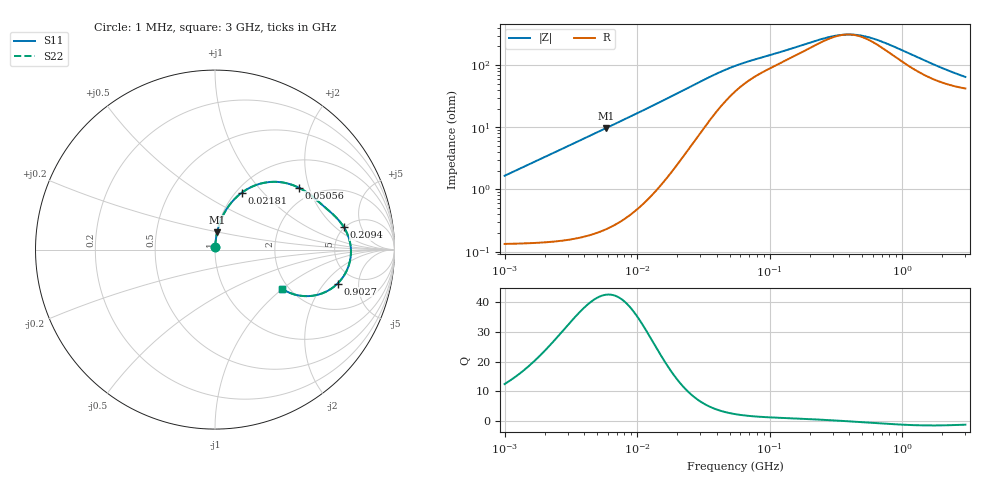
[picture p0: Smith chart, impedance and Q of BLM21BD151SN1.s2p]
! BLM21BD151SN1
# Hz S RI R 50
!Freq.(Hz) S11(Real) S11(Imag) S21(Real) S21(Imag) S12(Real) S12(Imag) S22(Real) S22(Imag)
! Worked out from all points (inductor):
!   401 points, 1 MHz to 3 GHz, reference 50 ohm
!   read as one part in series: L = 263 nH near 1.041 MHz
!   highest Q = 42.5 at 5.821 MHz (marker M1), where L = 265 nH
!   self-resonance near 385.4 MHz
!   S11 on the Smith chart (normalised r, x): 1 MHz: 1.00, +0.03; 21.81 MHz: 1.06, +0.77; 50.56 MHz: 1.64, +1.71; 209.4 MHz: 4.95, +2.62; 902.7 MHz: 3.65, -2.77; 3 GHz: 1.84, -0.98
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1000000  0.0016 0.0165  0.9984 -0.0165  0.9984 -0.0165  0.0016 0.0165
3823119  0.00568 0.0629  0.9943 -0.0629  0.9943 -0.0629  0.00568 0.0629
5820586  0.0115 0.0955  0.9885 -0.0955  0.9885 -0.0955  0.0115 0.0955
9410094  0.0283 0.1528  0.9717 -0.1528  0.9717 -0.1528  0.0283 0.1528
1.461624e7  0.0676 0.2305  0.9324 -0.2305  0.9324 -0.2305  0.0676 0.2305
2.181181e7  0.1484 0.3164  0.8516 -0.3164  0.8516 -0.3164  0.1484 0.3164
2.773354e7  0.2281 0.3596  0.7719 -0.3596  0.7719 -0.3596  0.2281 0.3596
3.387922e7  0.3094 0.377  0.6906 -0.377  0.6906 -0.377  0.3094 0.377
4.05666e7  0.3847 0.3727  0.6153 -0.3727  0.6153 -0.3727  0.3847 0.3727
5.055795e7  0.4654 0.3458  0.5346 -0.3458  0.5346 -0.3458  0.4654 0.3458
5.477226e7  0.4899 0.3325  0.5101 -0.3325  0.5101 -0.3325  0.4899 0.3325
8.679508e7  0.5896 0.256  0.4104 -0.256  0.4104 -0.256  0.5896 0.256
2.094008e8  0.7185 0.1239  0.2815 -0.1239  0.2815 -0.1239  0.7185 0.1239
3.124888e8  0.7511 0.0451  0.2489 -0.0451  0.2489 -0.0451  0.7511 0.0451
4.135554e8  0.7574 -0.0156  0.2426 0.0156  0.2426 0.0156  0.7574 -0.0156
5.473095e8  0.748 -0.0791  0.252 0.0791  0.252 0.0791  0.748 -0.0791
8.005644e8  0.7047 -0.1646  0.2953 0.1646  0.2953 0.1646  0.7047 -0.1646
9.0272e8  0.6827 -0.1893  0.3173 0.1893  0.3173 0.1893  0.6827 -0.1893
1.218836e9  0.6105 -0.2383  0.3895 0.2383  0.3895 0.2383  0.6105 -0.2383
1.613037e9  0.5293 -0.2587  0.4707 0.2587  0.4707 0.2587  0.5293 -0.2587
2.092429e9  0.4547 -0.253  0.5453 0.253  0.5453 0.253  0.4547 -0.253
3e9  0.3714 -0.2172  0.6286 0.2172  0.6286 0.2172  0.3714 -0.2172
